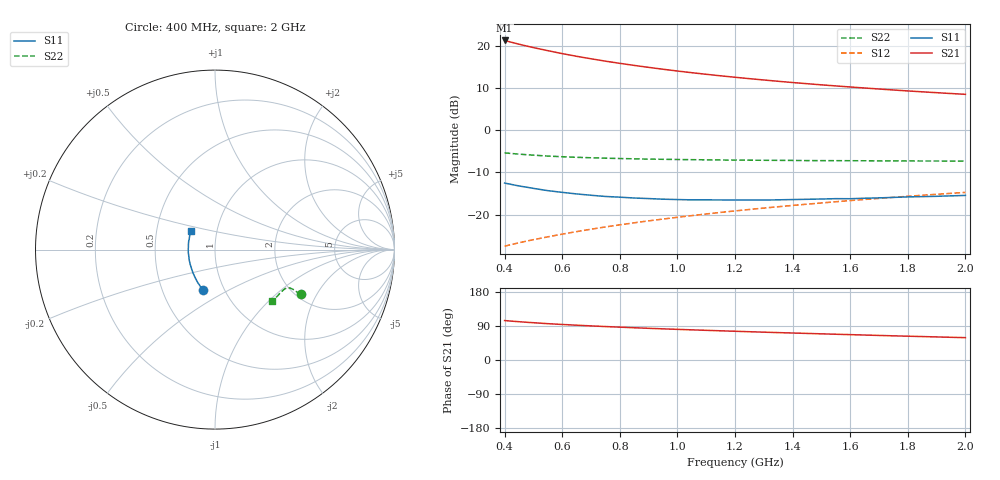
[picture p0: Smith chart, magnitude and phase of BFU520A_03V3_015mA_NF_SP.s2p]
! Filename:  P:\Prog\Test\Noise\ATS_data\Testdata_Net\06 Compressed Noise after Statistics\BFU520A_APG2013_30_A05_03p3V_015mA_NF_CM01_D.sf
! Date/Time: Wed 24/Apr/2013 20:06:17
! BFU520A_APG2013_30_A05_03p3V_1to20mA_NF_CM01_Bias7_R.sf
! Noise Parameter Data File
! BFU520A_APG2013_30_A05_03p3V_1to20mA_NF_CM01
! Date/time: Thu Apr 11 00:04:13 2013
! VAR V_out= 3.300000
! VAR I_out= 15.000000
! VAR V_in= 0.856500
! VAR I_in= 0.173300
! Device data file deembeded for feedlines and parallel
! Original file: \06 Compressed Noise after Statistics\BFU520A_APG2013_30_A05_03p3V_015mA_NF_CM01_R.sf
! Feed-files: PR017V01_150413_Feed1.s2p, PR017V01_150413_Feed2.s2p
! Parallel-file: PR017V01_150413_Par.s2p
# MHz S MA R 50
!  Freq-MHz  S11-mag  S11-arg  S21-mag  S21-arg  S12-mag  S12-arg  S22-mag  S22-arg
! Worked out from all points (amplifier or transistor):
!   37 points, 400 MHz to 2 GHz, reference 50 ohm
!   highest |S21| = 21.2 dB at 400 MHz (marker M1)
!   |S21| within 3 dB of that: start of sweep to 592 MHz
!   unconditionally stable (mu >= 1): 932.5 MHz to 1.873 GHz
!   at 500 MHz: K = 0.91, MSG = 22.7 dB, |S12| = -25.9 dB
!   at 1.1 GHz: K = 1.01, MAG = 16.0 dB, |S12| = -19.8 dB
!   at 2 GHz: K = 0.99, MSG = 11.6 dB, |S12| = -14.7 dB
!   lowest NFmin = 0.99 dB at 433 MHz
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400  0.2362 -105.8  11.48 104.1  0.0424 71.0  0.538 -27.6
420  0.229 -108.5  11.01 102.8  0.04405 71.2  0.53 -27.5
440  0.2218 -111.3  10.58 101.6  0.04567 71.4  0.523 -27.4
460  0.2156 -113.6  10.17 100.5  0.0473 71.6  0.5167 -27.4
480  0.2102 -116.2  9.797 99.4  0.04895 71.8  0.5103 -27.3
500  0.2045 -118.8  9.449 98.4  0.05058 72.0  0.5053 -27.2
550  0.1922 -124.8  8.695 95.9  0.05464 72.5  0.4928 -27.1
600  0.1835 -130.0  8.023 93.8  0.05883 72.8  0.4842 -27.0
650  0.1758 -135.1  7.46 91.8  0.06302 73.1  0.4766 -27.1
700  0.1696 -140.0  6.968 90.0  0.06727 73.4  0.4705 -27.1
750  0.1641 -144.8  6.534 88.3  0.07155 73.6  0.4653 -27.3
800  0.161 -149.2  6.156 86.7  0.07582 73.8  0.4612 -27.5
850  0.1573 -153.8  5.819 85.1  0.0801 73.8  0.4572 -27.8
950  0.1524 -161.8  5.241 82.2  0.08876 74.0  0.4515 -28.5
1050  0.1496 -169.1  4.772 79.6  0.09743 74.0  0.4467 -29.3
1150  0.1493 -176.2  4.384 77.0  0.1063 73.9  0.443 -30.3
1200  0.149 -179.3  4.214 75.8  0.1107 73.8  0.4419 -30.8
1350  0.1498 171.7  3.776 72.3  0.1241 73.3  0.4387 -32.5
1500  0.1531 163.7  3.428 69.0  0.1375 72.8  0.4352 -34.4
1600  0.1543 159.1  3.234 67.0  0.1467 72.4  0.4343 -35.9
1750  0.16 152.2  2.98 63.8  0.1603 71.7  0.4322 -38.0
2000  0.1688 142.6  2.647 59.0  0.1833 70.3  0.4301 -41.9
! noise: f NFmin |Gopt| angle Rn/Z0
400  1.022  0.1635  -160.7  0.0966
460  1.008  0.1827  -164.9  0.0857
600  1.093  0.1714  -155.9  0.1049
800  1.057  0.2029  -154.3  0.0884
1000  1.099  0.2185  -148.6  0.0895
1200  1.142  0.2187  -145.2  0.0958
1400  1.172  0.2539  -136.4  0.1004
1600  1.178  0.2712  -132.6  0.1034
1800  1.184  0.2959  -126.6  0.1076
2000  1.201  0.3104  -124.7  0.1155
